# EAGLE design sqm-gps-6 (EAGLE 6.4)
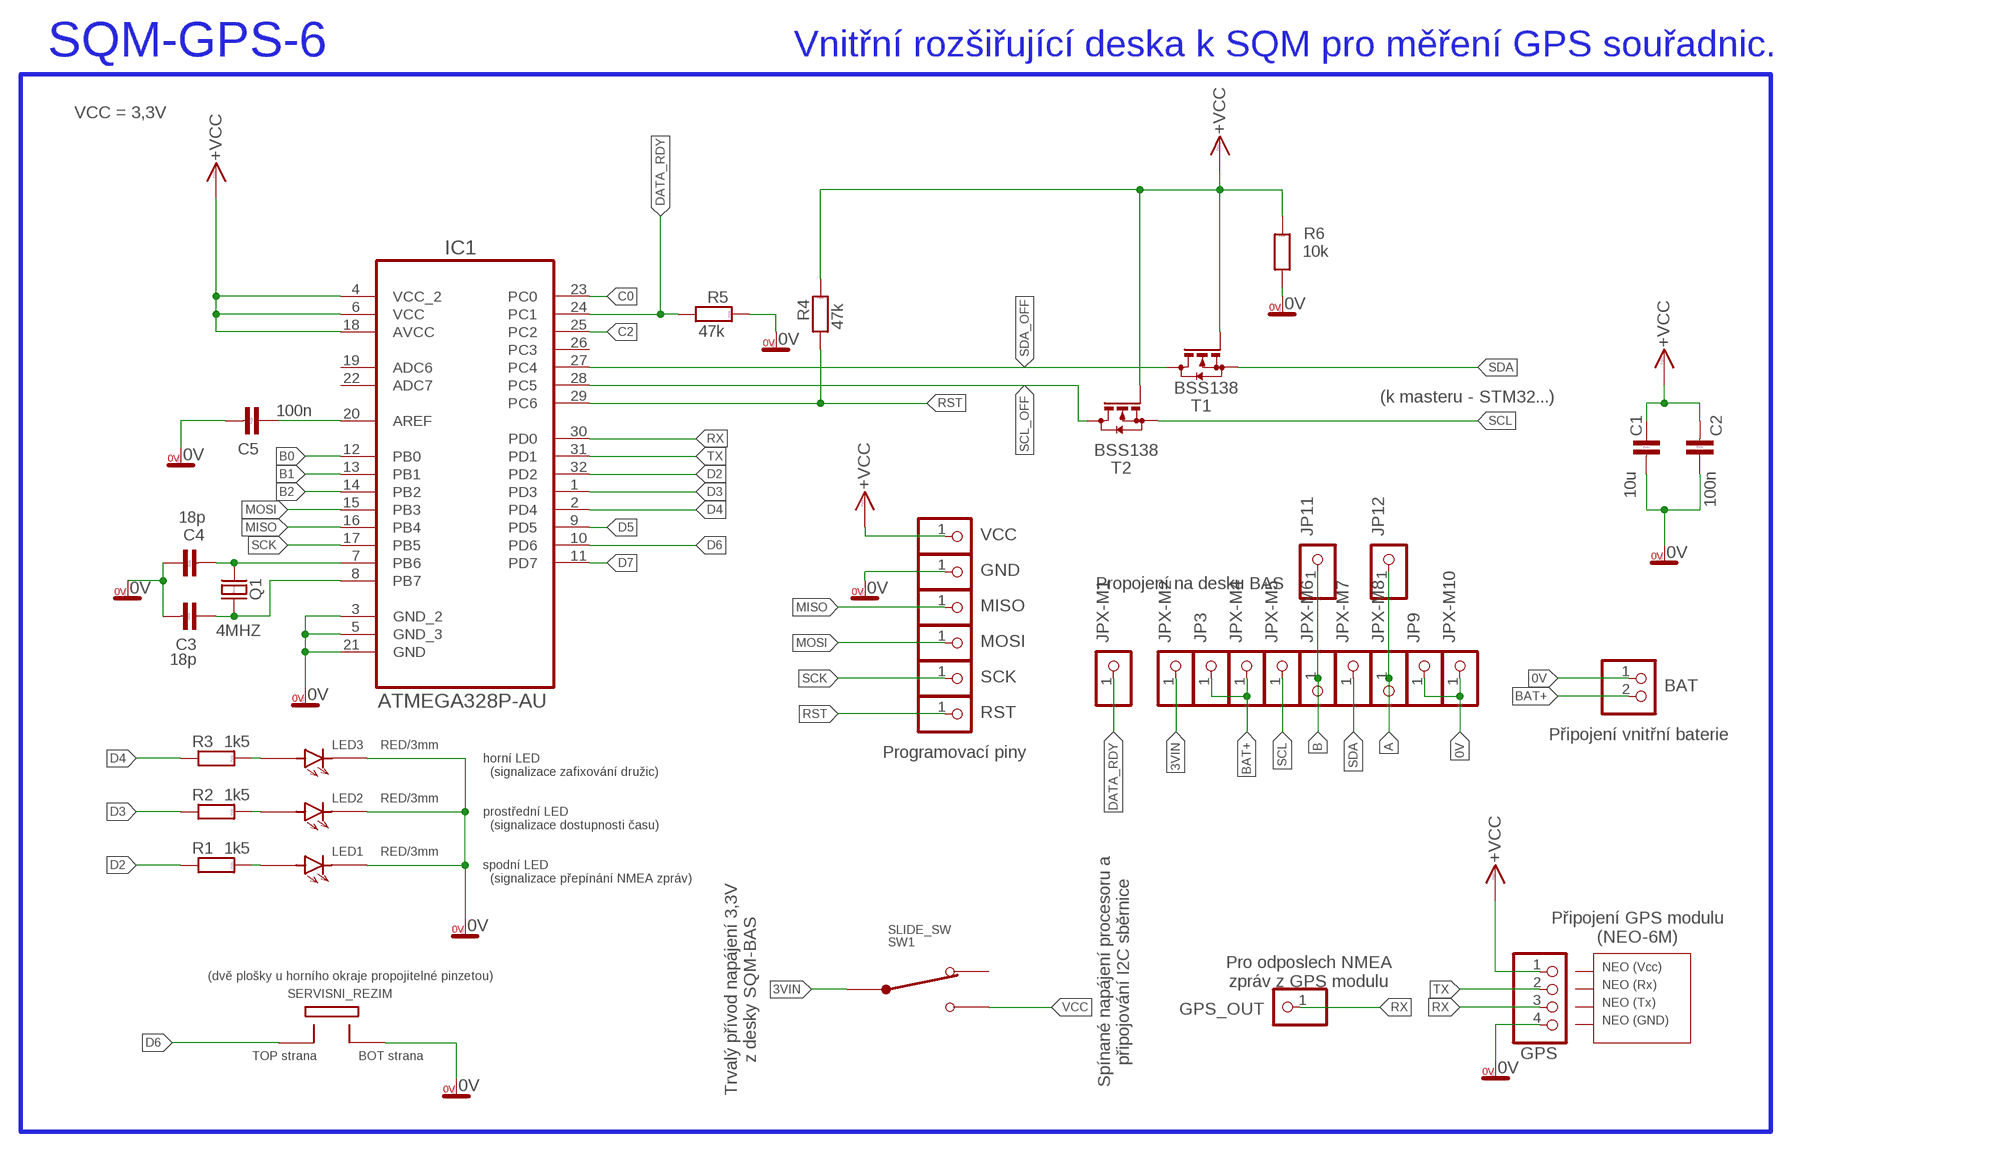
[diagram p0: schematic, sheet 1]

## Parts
BAT  PINHD-1X2  [1X02]
C1  10u  C-KERAMIK_SMD_1206  [1206]
C2  100n  C-KERAMIK_SMD_0805  [0805]
C3  18p  C-KERAMIK_SMD_0805  [0805]
C4  18p  C-KERAMIK_SMD_0805  [0805]
C5  100n  C-KERAMIK_SMD_0805  [0805]
GND  PINHD-1X1  [1X01]
GPS  PINHD-1X4  [1X04]
GPS_OUT  PINHD-1X1  [1X01]
IC1  ATMEGA328P-AU  [QFP80P900X900X120-32N]
JP3  PINHD-1X1  [1X01]
JP9  PINHD-1X1  [1X01]
JP11  PINHD-1X1  [1X01]
JP12  PINHD-1X1  [1X01]
JPX-M1  PINHD-1X1  [1X01]
JPX-M2  PINHD-1X1  [1X01]
JPX-M4  PINHD-1X1  [1X01]
JPX-M5  PINHD-1X1  [1X01]
JPX-M6  PINHD-1X1  [1X01]
JPX-M7  PINHD-1X1  [1X01]
JPX-M8  PINHD-1X1  [1X01]
JPX-M10  PINHD-1X1  [1X01]
LED1  RED/3mm  LED3MM_BOK  [LED3MM_BOK]
LED2  RED/3mm  LED3MM_BOK  [LED3MM_BOK]
LED3  RED/3mm  LED3MM_BOK  [LED3MM_BOK]
MISO  PINHD-1X1  [1X01]
MOSI  PINHD-1X1  [1X01]
Q1  4MHZ  Q_HC-49U  [HC-49U]
R1  1k5  R_SMD_0805  [0805]
R2  1k5  R_SMD_0805  [0805]
R3  1k5  R_SMD_0805  [0805]
R4  47k  R_SMD_0805  [0805]
R5  47k  R_SMD_0805  [0805]
R6  10k  R_SMD_0805  [0805]
RST  PINHD-1X1  [1X01]
SCK  PINHD-1X1  [1X01]
SERVISNI_REZIM  TOP_BOT_PIN  [TOP_BOT_PIN]
SW1  SLIDE_SW  [SLIDE_SW]
T1  BSS138  BSS123  [SOT23]
T2  BSS138  BSS123  [SOT23]
VCC  PINHD-1X1  [1X01]

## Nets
0V: BAT.1 C1.2 C2.1 C3.2 C4.1 C5.2 GND.1 GPS.4 IC1.3(GND_2) IC1.5(GND_3) IC1.21(GND) JP9.1 JPX-M10.1 LED1.K LED2.K LED3.K R5.2 R6.1 SERVISNI_REZIM.P2
3VIN: JPX-M2.1 SW1.PIN_COM
A: JP12.1 JPX-M8.1
AREF: C5.1 IC1.20(AREF)
B: JP11.1 JPX-M6.1
B0: IC1.12(PB0)
B1: IC1.13(PB1)
B2: IC1.14(PB2)
B6: C4.2 IC1.7(PB6) Q1.2
B7: C3.1 IC1.8(PB7) Q1.1
BAT+: BAT.2 JP3.1 JPX-M4.1
C0: IC1.23(PC0)
C2: IC1.25(PC2)
D2: IC1.32(PD2) R1.1
D3: IC1.1(PD3) R2.1
D4: IC1.2(PD4) R3.1
D5: IC1.9(PD5)
D6: IC1.10(PD6) SERVISNI_REZIM.P1
D7: IC1.11(PD7)
DATA_RDY: IC1.24(PC1) JPX-M1.1 R5.1
LED1_A1: LED1.A R1.2
LED2_A1: LED2.A R2.2
LED3_A1: LED3.A R3.2
MISO: IC1.16(PB4) MISO.1
MOSI: IC1.15(PB3) MOSI.1
RST: IC1.29(PC6) R4.1 RST.1
RX: GPS.3 GPS_OUT.1 IC1.30(PD0)
SCK: IC1.17(PB5) SCK.1
SCL: JPX-M5.1 T2.2(S)
SCL_OFF: IC1.28(PC5) T2.3(D)
SDA: JPX-M7.1 T1.2(S)
SDA_OFF: IC1.27(PC4) T1.3(D)
TX: GPS.2 IC1.31(PD1)
VCC: C1.1 C2.2 GPS.1 IC1.4(VCC_2) IC1.6(VCC) IC1.18(AVCC) R4.2 R6.2 SW1.PIN_2 T1.1(G) T2.1(G) VCC.1 ; supply symbol labelled +VCC
Unconnected: IC1.19(ADC6) IC1.22(ADC7) IC1.26(PC3) SW1.PIN_1

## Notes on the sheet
- SQM-GPS-6 | Vnitřní rozšiřující deska k SQM pro měření GPS souřadnic.
- VCC = 3,3V
- (k masteru - STM32...)
- Propojení na desku BAS
- Připojení vnitřní baterie
- Programovací piny
- horní LED
    (signalizace zafixování družic)
- prostřední LED
    (signalizace dostupnosti času)
- spodní LED
    (signalizace přepínání NMEA zpráv)
- Připojení GPS modulu
  (NEO-6M)
- Spínané napájení procesoru a
  připojování I2C sběrnice
- Pro odposlech NMEA
  zpráv z GPS modulu
- NEO (Vcc)
- (dvě plošky u horního okraje propojitelné pinzetou)
- Trvalý přívod napájení 3,3V
  z desky SQM-BAS
- NEO (Rx)
- NEO (Tx)
- NEO (GND)
- TOP strana | BOT strana

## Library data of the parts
BAT = pinhead:PINHD-1X2: PIN HEADER
C1-C5 = #PaJa_30:C-KERAMIK: Kondenzator - keramicky
GND GPS_OUT JP3 JP9 JP11 JP12 JPX-M1 JPX-M2 JPX-M4-JPX-M8 JPX-M10 MISO MOSI RST SCK VCC = pinhead:PINHD-1X1: PIN HEADER
GPS = pinhead:PINHD-1X4: PIN HEADER
IC1 = Atmel-ATMEGA328P-AU:ATMEGA328P-AU; DESCRIPTION: 8-bit Microcontroller with In-System Programmable Flash; MPN: ATMEGA328P-AU; OC_FARNELL: 1715486; OC_NEWARK: 14R4631; PACKAGE: TQFP-32; SUPPLIER: Atmel
LED1-LED3 = LED3mm_BOK:LED3MM_BOK: LED na okraji desky
Q1 = #PaJa_30:Q_HC-49U: Krystal - 1MHz - 48MHz
R1-R6 = #PaJa_30:R: Rezistor
SERVISNI_REZIM = TOP_BOT_PIN:TOP_BOT_PIN
SW1 = SLIDE_SW:SLIDE_SW: Posuvny prepinac
T1 T2 = transistor-small-signal:BSS123: N-CHANNEL MOS FET

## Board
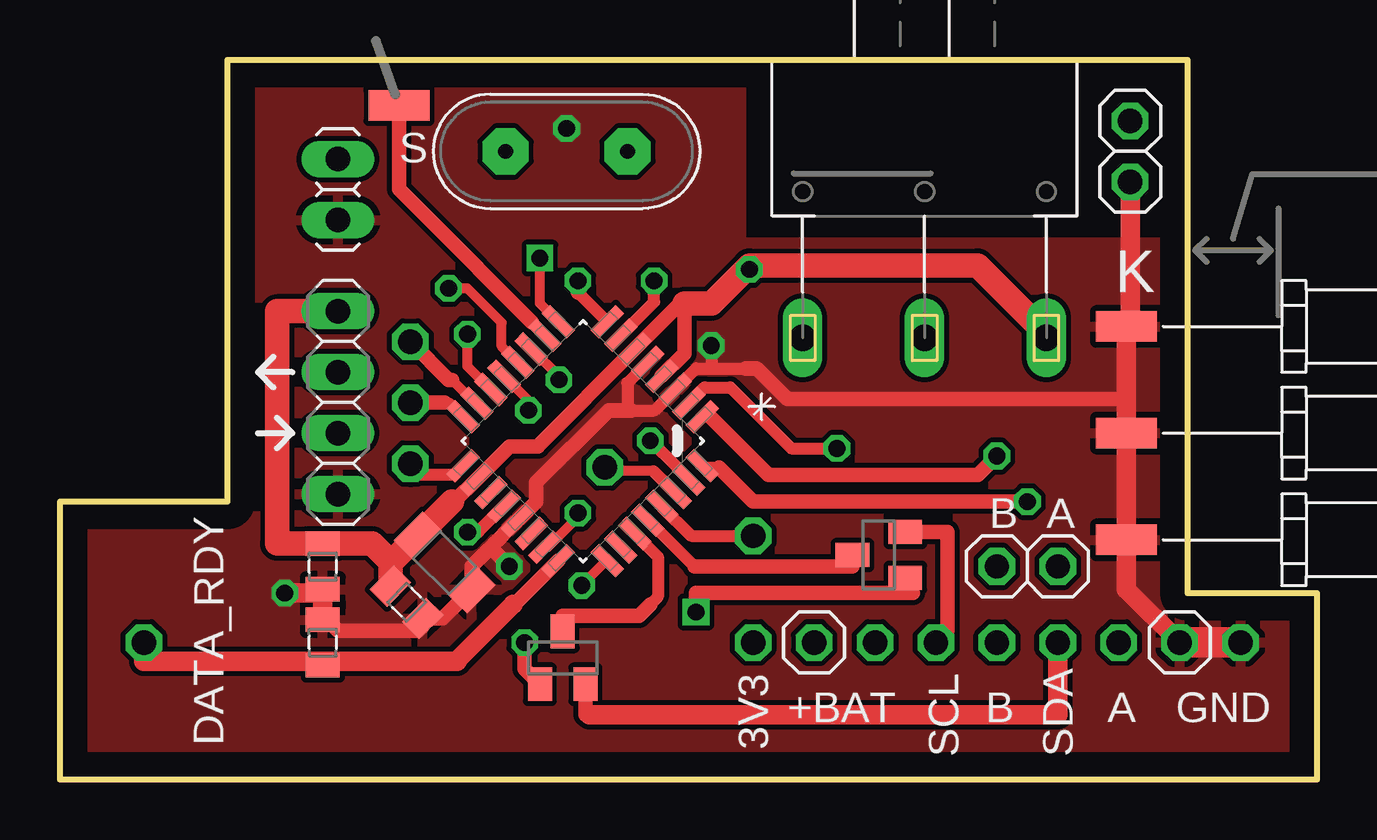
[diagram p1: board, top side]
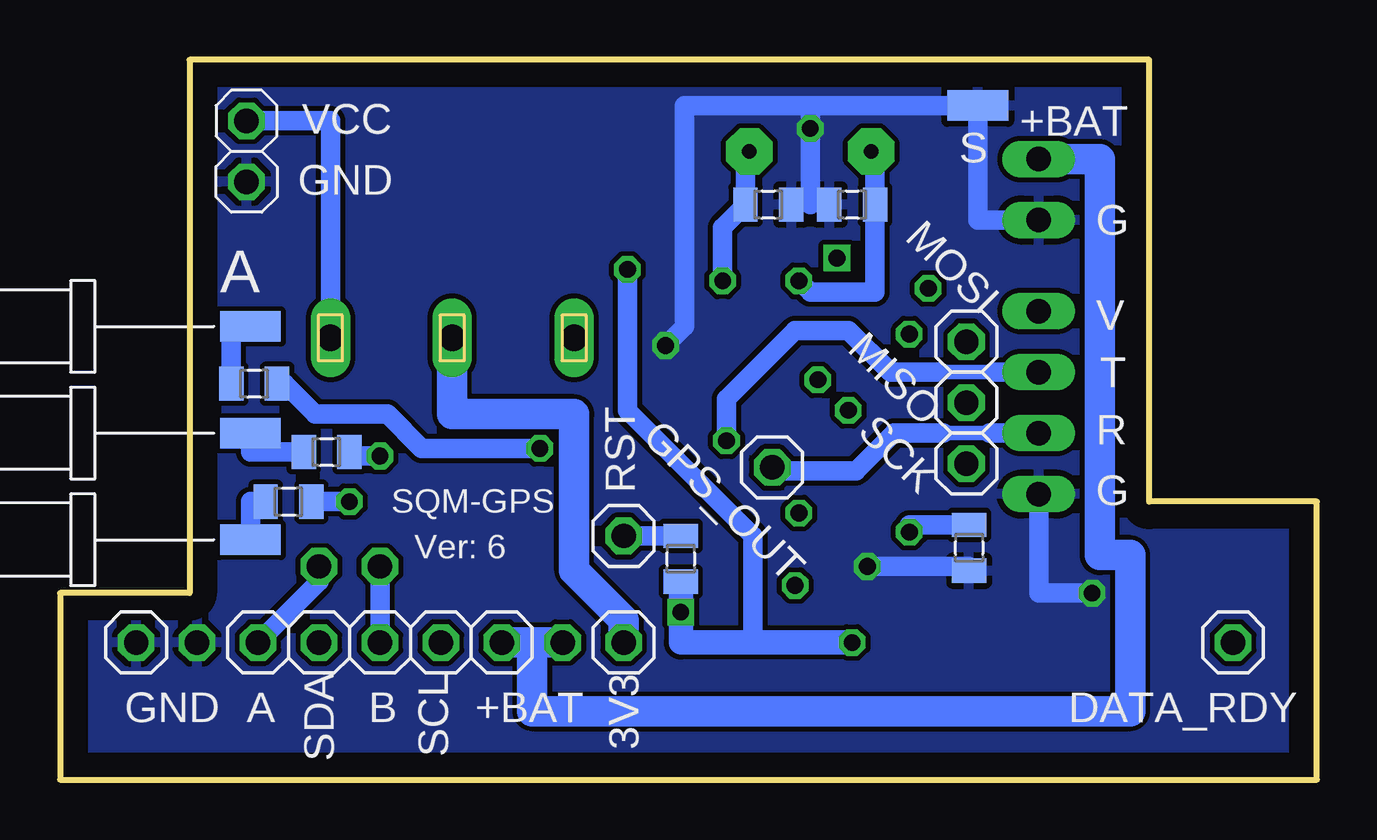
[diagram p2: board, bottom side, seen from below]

Size 52.39 x 30 mm. Coordinates in mm from the lower left corner, seen from the top.
Outline: 0,11.59 6.99,11.59 6.99,30 46.99,30 46.99,7.78 52.39,7.78 52.39,0 0,0 0,11.59
Copper layers (1*16): Top 0.035mm / dielectric 1.5mm / Bottom 0.035mm
Design rules "default *": minimum track width 10mil, minimum drill 24mil, track to track 8mil, track to pad 8mil, pad to pad 8mil, via to via 8mil, smd to smd 8mil, copper to edge 40mil, drill to drill 8mil, minimum pad ring 10mil, minimum via ring 8mil, stop-mask expansion 4mil, vias tented up to drill 0mil, thermal gap 10mil

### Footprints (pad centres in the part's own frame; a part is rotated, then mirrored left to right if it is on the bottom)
1X02 = drill 1.016 long: 1 -1.27,0; 2 1.27,0
1206 = smd 1.143 x 1.702: 1 -1.587,0; 2 1.587,0
0805 = smd 1.016 x 1.422: 1 -0.953,0; 2 0.953,0
1X01 = drill 1.016 octagon: 1 0,0
1X04 = drill 1.016 long: 1 -3.81,0; 2 -1.27,0; 3 1.27,0; 4 3.81,0
QFP80P900X900X120-32N = smd 1.473 x 0.508: 1 -4.242,2.794; 2 -4.242,2.007; 3 -4.242,1.194; 4 -4.242,0.406; 5 -4.242,-0.406; 6 -4.242,-1.194; 7 -4.242,-2.007; 8 -4.242,-2.794; 17 4.242,-2.794; 18 4.242,-2.007; 19 4.242,-1.194; 20 4.242,-0.406; 21 4.242,0.406; 22 4.242,1.194; 23 4.242,2.007; 24 4.242,2.794 | smd 0.508 x 1.473: 9 -2.794,-4.242; 10 -2.007,-4.242; 11 -1.194,-4.242; 12 -0.406,-4.242; 13 0.406,-4.242; 14 1.194,-4.242; 15 2.007,-4.242; 16 2.794,-4.242; 25 2.794,4.242; 26 2.007,4.242; 27 1.194,4.242; 28 0.406,4.242; 29 -0.406,4.242; 30 -1.194,4.242; 31 -2.007,4.242; 32 -2.794,4.242
LED3MM_BOK = smd 2.54 x 1.27 bottom: A 0,0 | smd 2.54 x 1.27: K 0,0
HC-49U = drill 0.61 pad 1.93 octagon: 1 -2.54,0; 2 2.54,0
TOP_BOT_PIN = smd 2.54 x 1.27: P1 0,0 | smd 2.54 x 1.27 bottom: P2 0,0
SLIDE_SW = drill 1.1 long: PIN_1 -5.08,-7.62; PIN_2 5.08,-7.62; PIN_COM 0,-7.62
SOT23 = smd 1 x 1.4: 1 -0.95,-1.1; 2 0.95,-1.1; 3 0,1.1

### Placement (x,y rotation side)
BAT  11.59,24.61 90 top
C1  16.03,9.05 315 top
C2  14.45,7.4 135 top
C3  19.37,23.97 180 bottom
C4  22.86,23.97 180 bottom
C5  14.49,9.66 270 bottom
GND  44.61,24.92 0 top
GPS  11.59,15.72 270 top
GPS_OUT  22.7,13.02 0 bottom
IC1  21.8,14.11 225 top
JP3  31.43,5.71 0 top
JP9  46.67,5.71 0 top
JP11  39.05,8.89 0 top
JP12  41.59,8.89 0 top
JPX-M1  3.49,5.71 0 bottom
JPX-M2  28.89,5.71 0 bottom
JPX-M4  33.97,5.71 0 bottom
JPX-M5  36.51,5.71 0 bottom
JPX-M6  39.05,5.71 0 bottom
JPX-M7  41.59,5.71 0 bottom
JPX-M8  44.13,5.71 0 bottom
JPX-M10  49.21,5.71 0 bottom
LED1  44.45,10 0 top
LED2  44.45,14.45 0 top
LED3  44.45,18.89 0 top
MISO  14.61,15.72 0 bottom
MOSI  14.61,18.26 0 bottom
Q1  21.11,26.19 0 top
R1  42.86,11.59 180 bottom
R2  41.27,13.65 180 bottom
R3  44.29,16.51 180 bottom
R4  26.51,9.21 270 bottom
R5  10.95,5.71 90 top
R6  10.95,8.89 90 top
RST  28.89,10.16 0 bottom
SCK  14.61,13.18 0 bottom
SERVISNI_REZIM  14.13,28.1 180 top
SW1  36.04,26.04 0 top
T1  20.95,5.08 0 top
T2  34.13,9.37 90 top
VCC  44.61,27.46 0 top

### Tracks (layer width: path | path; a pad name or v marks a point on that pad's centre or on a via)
0V  (via drill 0.7)
  Top 0.406: IC1.21 18.9,10.64
  Top 0.508: 23.81,15.4 24.77,15.4 IC1.3 26.52,17.14 27.15,17.14 | 23.65,15.4 23.65,16.54 IC1.5 | 27.15,17.14 28.57,17.14 | v27.15,18.1 27.15,17.14
  Top 0.61: LED2.K 44.45,15.88 30.32,15.88 29.05,17.14 28.57,17.14 | 18.9,10.64 19.84,11.58 19.84,12.38 22.86,15.4 23.02,15.4 23.65,15.4 23.81,15.4 | 11.11,6.67 11.59,6.19 14.92,6.19 15.12,6.39 C2.1 15.95,6.72 C1.2 17.16,8.9 17.86,9.6 | IC1.21 17.86,9.6 | v18.73,8.89 18.02,9.6 17.86,9.6
  Top 0.813: JP9.1 44.45,7.94 LED1.K LED2.K LED3.K 44.61,18.89 GND.1 | 10.95,7.78 R5.2 11.11,6.67 | 10.95,7.78 R6.1 | v9.37,7.78 10.95,7.78
  Top 1.27: JP9.1 JPX-M10.1
  Bottom 0.61: C3.2 21.11,23.97 C4.1
  Bottom 0.813: 21.11,28.1 SERVISNI_REZIM.P2 14.13,23.34 BAT.1 | 21.11,28.1 v21.11,27.15 21.11,23.97 | 21.11,28.1 26.35,28.1 26.35,18.89 v27.15,18.1 | C5.2 14.49,8.89 v18.73,8.89 | GPS.4 11.59,7.78 v9.37,7.78
  pour Top: 6.99,11.59 0,11.59 0,0 52.39,0 52.39,7.78 46.99,7.78 46.99,22.38 28.42,22.38 28.42,30 6.99,30
  pour Bottom: 6.99,30 46.99,30 46.99,7.78 52.39,7.78 52.39,0 0,0 0,11.59 6.99,11.59
3VIN
  Bottom 0.813: 30.96,14.29 30.96,15.24
  Bottom 1.27: SW1.PIN_COM 36.04,15.24 30.96,15.24 30.96,8.73 28.89,6.67 JPX-M2.1
A
  Bottom 0.813: JPX-M8.1 41.59,8.26 JP12.1
AREF  (via drill 0.7)
  Top 0.508: IC1.20 17.43,10.32 v16.99,10.32
  Bottom 0.813: v16.99,10.32 16.99,10.62 C5.1
B
  Bottom 0.813: JPX-M6.1 JP11.1
B0  (via drill 0.7)
  Top 0.406: IC1.12 18.41,18.06 18.41,19.05 16.99,20.48 v16.19,20.48
B1  (via drill 0.7)
  Top 0.406: IC1.13 19.53,15.8 v19.53,15.4
B2  (via drill 0.7)
  Top 0.406: IC1.14 16.99,17.23 v16.99,18.57
B6  (via drill 0.7)
  Top 0.508: IC1.7 24.77,19.92 v24.77,20.8
  Bottom 0.813: Q1.2 23.81,26.19 C4.2 24.77,23.02 v24.77,20.8
B7  (via drill 0.7)
  Top 0.508: 21.59,20.31 IC1.8
  Top 0.61: v21.59,20.8 21.59,20.31
  Bottom 0.813: Q1.1 18.41,26.19 C3.1 18.41,20.32 21.11,20.32 v21.59,20.8
BAT+
  Bottom 1.27: BAT.2 9.05,25.88 9.05,9.37 7.78,9.37 7.78,2.86 32.7,2.86 32.7,5.71 JPX-M4.1 JP3.1
C0  (via drill 0.7)
  Top 0.406: IC1.23 20.33,9.69 21.59,10.95 v21.59,11.11
C2  (via drill 0.7)
  Top 0.406: IC1.25 22.79,9.13 v21.75,8.1
D2  (via drill 0.7)
  Top 0.406: IC1.32 26.84,13.02
  Top 0.508: 26.84,13.02 27.46,13.02
  Top 0.61: v40.32,11.59 28.89,11.59 27.46,13.02
  Bottom 0.813: v40.32,11.59 R1.1
D3  (via drill 0.7)
  Top 0.406: 26.99,15.24 26.88,15.13 IC1.1 27.09,15.13
  Top 0.61: 27.09,15.13 29.53,12.7 38.26,12.7 v39.05,13.49
  Bottom 0.813: v39.05,13.49 40.32,13.49 R2.1
D4  (via drill 0.7)
  Top 0.508: IC1.2 26.88,16.35 27.94,16.35 30.48,13.81 v32.38,13.81
  Bottom 0.813: v32.38,13.81 37.31,13.81 38.73,15.24 41.75,15.24 43.02,16.51 R3.1
D5  (via drill 0.7)
  Top 0.406: IC1.9 20,19.85 v20,21.75
D6
  Top 0.406: 19.84,18.89 19.68,19.05 | 15.88,22.86 | IC1.10 18.98,19.76 18.97,19.76
  Top 0.61: 19.68,19.05 18.97,19.76 15.88,22.86 | 15.88,22.86 14.13,24.61 SERVISNI_REZIM.P1
D7  (via drill 0.7)
  Top 0.406: 19.68,17.94 20.8,16.83 v20.8,16.67 20.8,16.8 IC1.11
DATA_RDY
  Top 0.508: IC1.24 19.84,8.21
  Top 0.61: 16.56,4.92 IC1.24 | IC1.24
  Top 0.813: 10.95,4.92 3.49,4.92 JPX-M1.1 | R5.1 10.95,4.92 | 10.95,4.92 16.51,4.92 | 16.51,4.92 16.56,4.92 | 16.51,4.92 18.89,7.3
LED1_A1
  Bottom 0.813: R1.2 44.45,11.59 LED1.A
LED2_A1
  Bottom 0.813: R2.2 44.45,13.65 LED2.A
LED3_A1
  Bottom 0.813: R3.2 45.24,18.89 LED3.A
MISO
  Top 0.406: 15.44,15.72 MISO.1 | IC1.16 16.24,15.72 16.03,15.72
  Top 0.61: 16.03,15.72 MISO.1
MOSI
  Top 0.406: IC1.15 17.33,15.69 16.35,16.67
  Top 0.61: 16.35,16.67 16.19,16.67 MOSI.1
RST
  Top 0.508: IC1.29 26.32,10.16 RST.1
  Bottom 0.813: R4.1 RST.1
RX
  Top 0.406: 24.73,12.86 22.7,12.86 GPS_OUT.1
  Top 0.508: IC1.30 24.73,12.86
  Bottom 0.61: 13.65,14.45 15.56,14.45
  Bottom 0.813: GPS.3 13.65,14.45 | 15.56,14.45 17.62,14.45 19.21,12.86 22.7,12.86 GPS_OUT.1
SCK
  Top 0.406: IC1.17 16.43,12.7
  Top 0.508: 16.43,12.7 14.61,12.7
  Top 0.61: 14.61,12.7 SCK.1
SCL
  Top 0.61: T2.2 36.99,10.32 36.99,7.46 36.99,6.19 JPX-M5.1
SCL_OFF
  Top 0.508: IC1.28 26.44,8.89
  Top 0.61: 26.44,8.89 31.43,8.89 32.87,8.89 33.03,8.89 T2.3
SDA
  Top 0.61: T1.2 21.91,2.7 22.07,2.7
  Top 0.813: 22.07,2.7 41.59,2.7 JPX-M7.1
SDA_OFF
  Top 0.508: IC1.27 24.92,9.29 24.92,7.62 24.61,7.3
  Top 0.61: T1.3 20.95,6.83 24.13,6.83 24.61,7.3
TX  (via drill 0.7)
  Top 0.406: 25.09,13.65 25.08,13.65
  Top 0.508: IC1.31 25.09,13.65 | v24.61,14.13 25.08,13.65
  Bottom 0.61: 13.49,16.99 15.72,16.99
  Bottom 0.813: GPS.2 13.49,16.99 | 15.72,16.99 17.78,16.99 19.53,18.73 21.75,18.73 24.61,15.88 v24.61,14.13
VCC  (via drill 0.7)
  Top 0.61: 26.04,19.84 26.04,17.77 IC1.4 | 16.35,11.59 16.44,11.59 IC1.18 18.73,13.88 19.92,13.88 19.92,13.92 IC1.6 25.84,19.84 27.15,19.84 | T1.1 19.37,4.62 v19.37,5.71 | 35.23,7.78 26.51,7.78 v26.51,6.99 | T2.1 35.23,7.78 | 35.23,7.78 35.55,7.78
  Top 0.813: C2.2 13.65,8.07 | 41.12,18.57 SW1.PIN_2 | v28.73,21.27 28.73,21.43 | R6.2 10.96,9.85 13.02,9.85
  Top 1.016: 11.11,9.85 13.02,9.85 13.02,9.84 13.8,9.06 | 16.35,11.59 14.93,10.17 C1.1 13.8,9.06 | 26.04,19.84 27.15,19.84 28.73,21.43 38.26,21.43 41.12,18.57 | GPS.1 9.05,19.53 9.05,9.84 R6.2 | 13.8,9.06 13.77,9.03 C2.2
  Bottom 0.61: 26.51,5.71 26.67,5.71
  Bottom 0.813: VCC.1 41.12,27.46 SW1.PIN_2 | v19.37,5.71 23.5,5.71 23.5,10.16 28.73,15.4 v28.73,21.27
  Bottom 1.016: R4.2 v26.51,6.99 26.51,5.71 v19.37,5.71

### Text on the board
tPlace: S | K | B | A | 3V3 | SCL | +BAT | B | A | GND | DATA_RDY | SDA
bPlace: +BAT | S | G | MOSI | A | V | MISO | T | RST | R | SCK | G | SQM-GPS | Ver: 6 | DATA_RDY | 3V3 | SCL | SDA | +BAT | B | A | GND
tDocu: Vnitřní deska GPS (ver. 6) pro SQM / TOP strana | OFF | ON | LED osadit 3mm nad / hranu plošného spoje
bDocu: Vnitřní deska GPS (ver. 6) pro SQM / BOT strana | D5 | B0 | B2 | D7 | B1 | C0 | C2 | Pro piny JP-M je možné použít 90° kolíkovou lištu, / ze které se odstraní některé piny. | Pin JP1 musí být osazen samostatně / (plast mezi JP1 a JP2 by překážel obvodu AP1501 na desce SQM-BAS). | Programovací piny (MISO / MOSI / SCK / RST / VCC / GND) / se po naprogramování procesoru odstraní.

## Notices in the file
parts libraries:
Copyright (C) PaJa 2001-2011
